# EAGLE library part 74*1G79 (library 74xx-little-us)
Single Positive-Edge-Triggered D-Type Flip-Flop Source: http://focus.ti.com/lit/ds/symlink/sn74lvc2g79.pdf
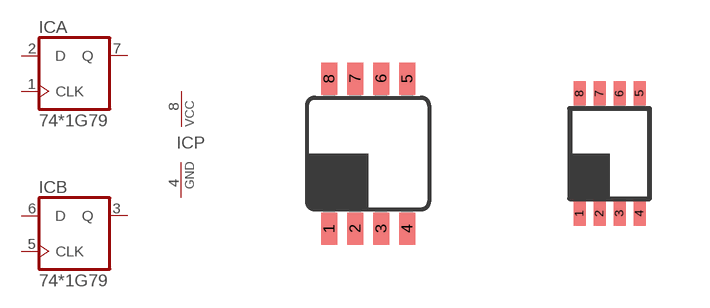
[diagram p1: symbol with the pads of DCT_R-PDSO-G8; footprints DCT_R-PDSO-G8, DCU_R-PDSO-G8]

Designator prefix IC; gates A=7479 P=PWRN B=7479

## 741G79DCT  [DCT_R-PDSO-G8]
1  A:CLK  in
2  A:D  in
3  B:Q  out
4  P:GND  pwr
5  B:CLK  in
6  B:D  in
7  A:Q  out
8  P:VCC  pwr

## 741G79DCU  [DCU_R-PDSO-G8]
Pads as for DCT_R-PDSO-G8

## 741G79YEP  [YEP_R-XBGA-N8]
A1  A:CLK  in
A2  P:VCC  pwr
B1  A:D  in
B2  A:Q  out
C1  B:Q  out
C2  B:D  in
D1  P:GND  pwr
D2  B:CLK  in

## Footprint DCT_R-PDSO-G8 (pad centres in mm)
DCT (R-PDSO-G8) PLSTIG SMALL-OUTLINE PACKAGE Source: http://focus.ti.com/lit/ds/symlink/sn74lvc2g53.pdf
smd 0.4 x 0.8: 1 -0.975,-1.875; 2 -0.325,-1.875; 3 0.325,-1.875; 4 0.975,-1.875; 5 0.975,1.875; 6 0.325,1.875; 7 -0.325,1.875; 8 -0.975,1.875

## Footprint DCU_R-PDSO-G8 (pad centres in mm)
DCU (R-PDSO-G8) PLASTIC SMALL-OUTLINE PACKAGE (DIE DOWN) Source: http://focus.ti.com/lit/ds/symlink/sn74lvc2g53.pdf
smd 0.3 x 0.6: 1 -0.75,-1.5; 2 -0.25,-1.5; 3 0.25,-1.5; 4 0.75,-1.5; 5 0.75,1.5; 6 0.25,1.5; 7 -0.25,1.5; 8 -0.75,1.5

## Footprint YEP_R-XBGA-N8 (pad centres in mm)
YEP (R-XBGA-N8) DIE-SIZE BALL GRID ARRAY Source: http://focus.ti.com/lit/ds/symlink/sn74lvc2g53.pdf
smd 0.3 x 0.3: A1 -0.75,-0.25; A2 -0.75,0.25; B1 -0.25,-0.25; B2 -0.25,0.25; C1 0.25,-0.25; C2 0.25,0.25; D1 0.75,-0.25; D2 0.75,0.25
